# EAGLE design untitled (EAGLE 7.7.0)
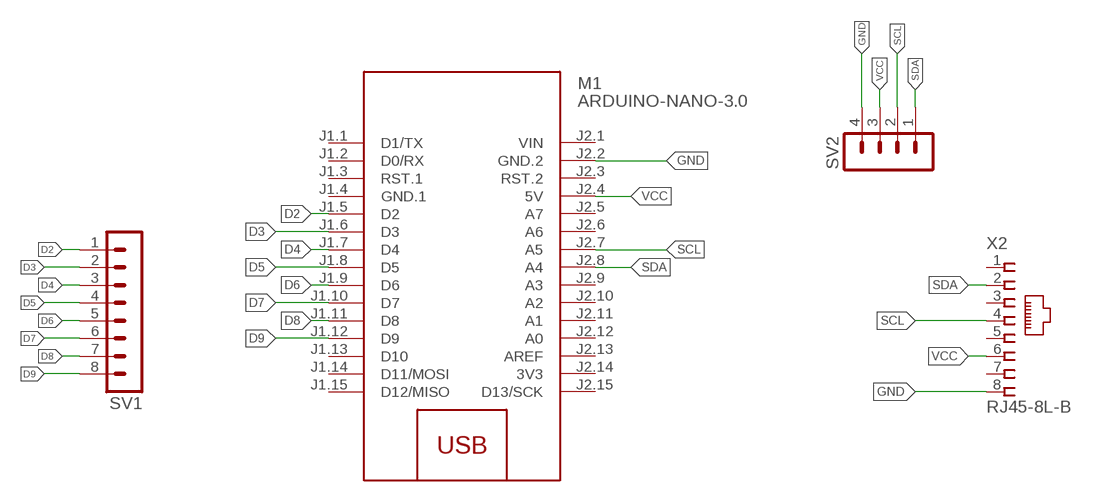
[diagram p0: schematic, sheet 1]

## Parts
M1  ARDUINO-NANO-3.0  [ARDUINO-NANO-3.0]
SV1  MA08-1  [MA08-1]
SV2  MA04-1  [MA04-1]
X2  RJ45-8L-B  [RJ45-NO-SHIELD]

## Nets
D2: M1.J1.5(D2) SV1.1
D3: M1.J1.6(D3) SV1.2
D4: M1.J1.7(D4) SV1.3
D5: M1.J1.8(D5) SV1.4
D6: M1.J1.9(D6) SV1.5
D7: M1.J1.10(D7) SV1.6
D8: M1.J1.11(D8) SV1.7
D9: M1.J1.12(D9) SV1.8
GND: M1.J2.2(GND.2) SV2.4 X2.8
SCL: M1.J2.7(A5) SV2.2 X2.4
SDA: M1.J2.8(A4) SV2.1 X2.2
VCC: M1.J2.4(5V) SV2.3 X2.6
Unconnected: M1.J1.1(D1/TX) M1.J1.2(D0/RX) M1.J1.3(RST.1) M1.J1.13(D10) M1.J1.14(D11/MOSI) M1.J1.15(D12/MISO) M1.J2.3(RST.2) M1.J2.5(A7) M1.J2.6(A6) M1.J2.9(A3) M1.J2.10(A2) M1.J2.11(A1) M1.J2.12(A0) M1.J2.13(AREF) M1.J2.15(D13/SCK) X2.1 X2.3 X2.5 X2.7

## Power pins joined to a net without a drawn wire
3V3: M1.J2.14(3V3)
GND.1: M1.J1.4(GND.1)
VIN: M1.J2.1(VIN)

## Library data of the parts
M1 = diy-modules:ARDUINO-NANO-3.0: Arduino Nano 3.0 and compatible devices More details available here: https://www.arduino.cc/en/Main/ArduinoBoardNano Click here to find device on ebay.com
SV1 = con-lstb:MA08-1: PIN HEADER; OC_FARNELL: unknown; OC_NEWARK: unknown
SV2 = con-lstb:MA04-1: PIN HEADER; OC_FARNELL: unknown; OC_NEWARK: unknown
X2 = con-tycoelectronics:RJ45: CORCOM Modular RJ Jacks No Shield Source: www.tycoelectronics.com .. ENG_DS_1654001_1099_RJ_L_0507.pdf; MF: TYCO ELECTRONICS; MPN: RJ45-8L-B; OC_FARNELL: 1279843; OC_NEWARK: 52K4445

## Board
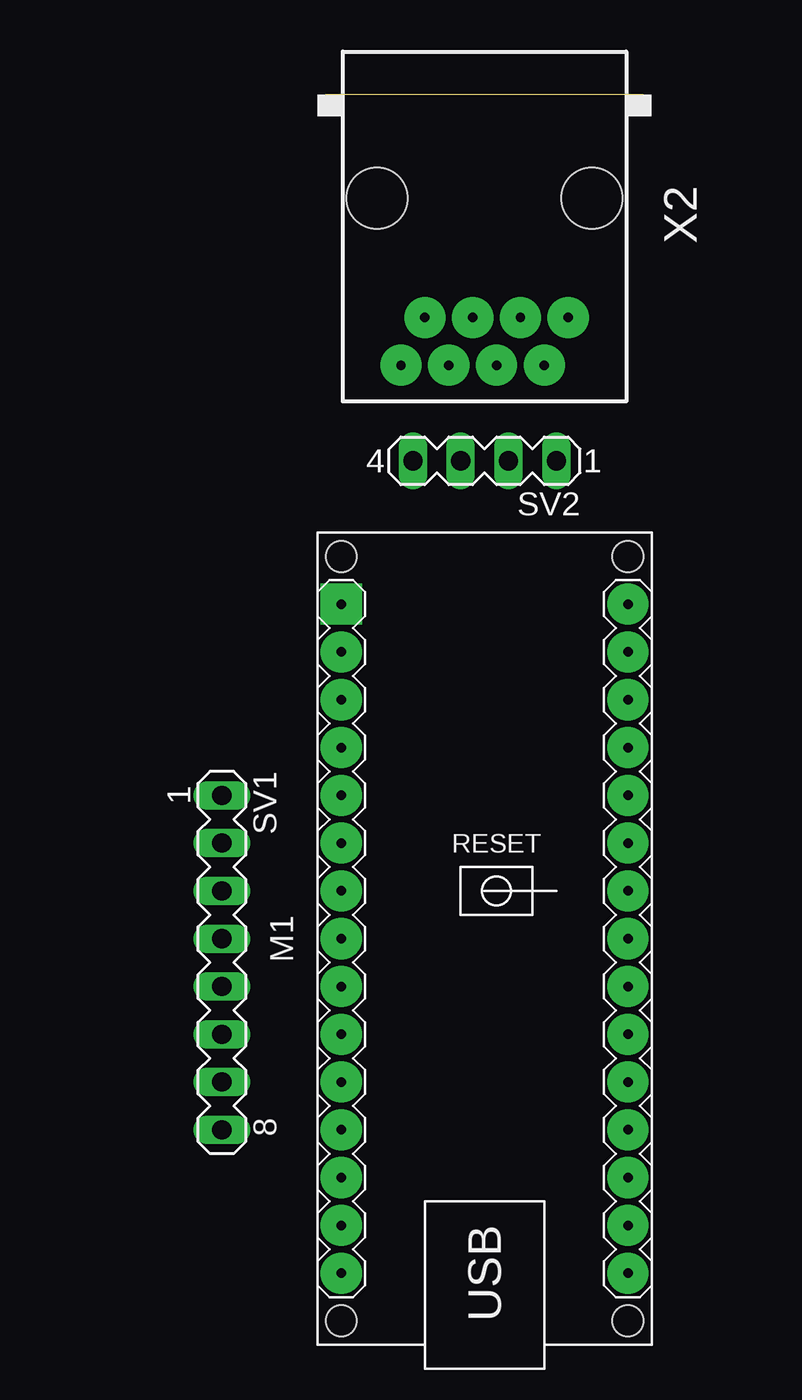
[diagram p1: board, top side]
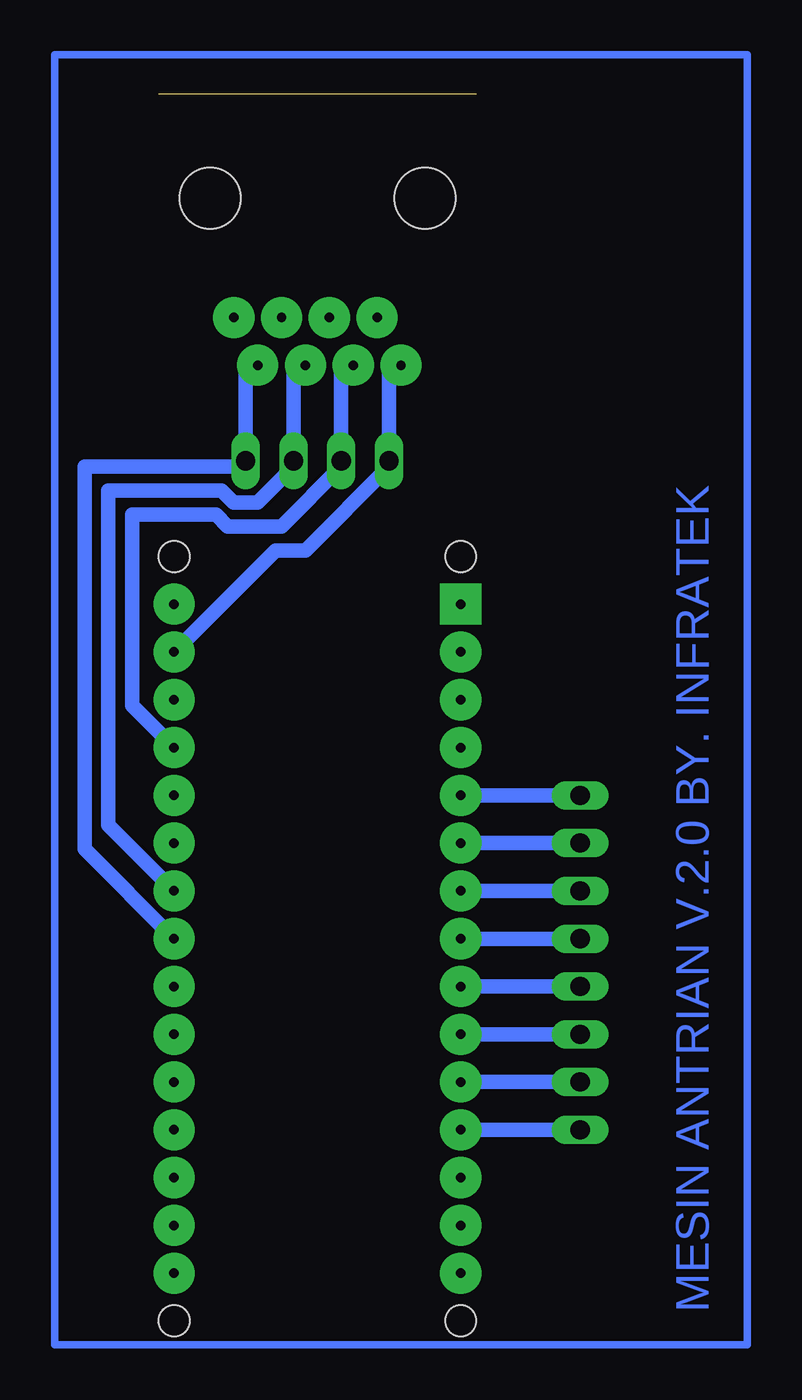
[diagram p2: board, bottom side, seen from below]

Size 16.89 x 0 mm. Coordinates in mm from the lower left corner, seen from the top.
Copper layers (1*16): Top 0.035mm / dielectric 1.5mm / Bottom 0.035mm
Design rules "default *": minimum track width 30mil, minimum drill 24mil, track to track 8mil, track to pad 8mil, pad to pad 8mil, via to via 8mil, smd to smd 8mil, copper to edge 40mil, drill to drill 8mil, minimum pad ring 10mil, minimum via ring 8mil, stop-mask expansion 4mil, vias tented up to drill 0mil, thermal gap 10mil

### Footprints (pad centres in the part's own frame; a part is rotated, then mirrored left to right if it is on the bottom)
ARDUINO-NANO-3.0 = drill 0.5 pad 2.184 square: J1.1 17.78,7.62 | drill 0.5 pad 2.184: J1.2 15.24,7.62; J1.3 12.7,7.62; J1.4 10.16,7.62; J1.5 7.62,7.62; J1.6 5.08,7.62; J1.7 2.54,7.62; J1.8 0,7.62; J1.9 -2.54,7.62; J1.10 -5.08,7.62; J1.11 -7.62,7.62; J1.12 -10.16,7.62; J1.13 -12.7,7.62; J1.14 -15.24,7.62; J1.15 -17.78,7.62; J2.1 17.78,-7.62; J2.2 15.24,-7.62; J2.3 12.7,-7.62; J2.4 10.16,-7.62; J2.5 7.62,-7.62; J2.6 5.08,-7.62; J2.7 2.54,-7.62; J2.8 0,-7.62; J2.9 -2.54,-7.62; J2.10 -5.08,-7.62; J2.11 -7.62,-7.62; J2.12 -10.16,-7.62; J2.13 -12.7,-7.62; J2.14 -15.24,-7.62; J2.15 -17.78,-7.62 | hole 1.651: -20.32,7.62; -20.32,-7.62; 20.32,-7.62; 20.32,7.62
MA08-1 = drill 1.016 long: 1 -8.89,0; 2 -6.35,0; 3 -3.81,0; 4 -1.27,0; 5 1.27,0; 6 3.81,0; 7 6.35,0; 8 8.89,0
MA04-1 = drill 1.016 long: 1 -3.81,0; 2 -1.27,0; 3 1.27,0; 4 3.81,0
RJ45-NO-SHIELD = drill 0.5 pad 2.184: 1 -4.445,6.35; 2 -3.175,8.89; 3 -1.905,6.35; 4 -0.635,8.89; 5 0.635,6.35; 6 1.905,8.89; 7 3.175,6.35; 8 4.445,8.89 | hole 3.251: -5.715,0; 5.715,0

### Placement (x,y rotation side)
M1  8.45,-44.88 90 top  (outside the outline)
SV1  -5.52,-46.15 270 top  (outside the outline)
SV2  8.45,-19.48 180 top  (outside the outline)
X2  8.45,-5.51 180 top  (outside the outline)

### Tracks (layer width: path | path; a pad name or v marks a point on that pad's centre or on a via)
D2
  Bottom 0.762: M1.J1.5 SV1.1
D3
  Bottom 0.762: M1.J1.6 SV1.2
D4
  Bottom 0.762: M1.J1.7 SV1.3
D5
  Bottom 0.762: M1.J1.8 SV1.4
D6
  Bottom 0.762: M1.J1.9 SV1.5
D7
  Bottom 0.762: M1.J1.10 SV1.6
D8
  Bottom 0.762: M1.J1.11 SV1.7
D9
  Bottom 0.762: M1.J1.12 SV1.8
GND
  Bottom 0.762: X2.8 4.64,-14.4 SV2.4 4.64,-19.8 9.08,-24.24 10.67,-24.24 M1.J2.2
N$1
  Bottom 0.406: -14.41,2.11 -14.41,-66.47 22.42,-66.47 22.42,2.11 -14.41,2.11
SCL
  Bottom 0.762: X2.4 9.72,-14.4 SV2.2 9.72,-19.8 11.62,-21.7 12.89,-21.7 13.53,-21.07 19.56,-21.07 19.56,-38.85 M1.J2.7
SDA
  Bottom 0.762: X2.2 12.26,-14.4 SV2.1 12.26,-19.8 20.83,-19.8 20.83,-40.12 M1.J2.8
VCC
  Bottom 0.762: X2.6 7.18,-14.4 SV2.3 7.18,-19.8 10.35,-22.97 13.21,-22.97 13.84,-22.34 18.29,-22.34 18.29,-32.5 M1.J2.4

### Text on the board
Bottom: MESIN ANTRIAN V.2.0 BY. INFRATEK

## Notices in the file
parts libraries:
diy-modules: Released under the Creative Commons Attribution 4.0 International License: http://creativecommons.org/licenses/by/4.0
